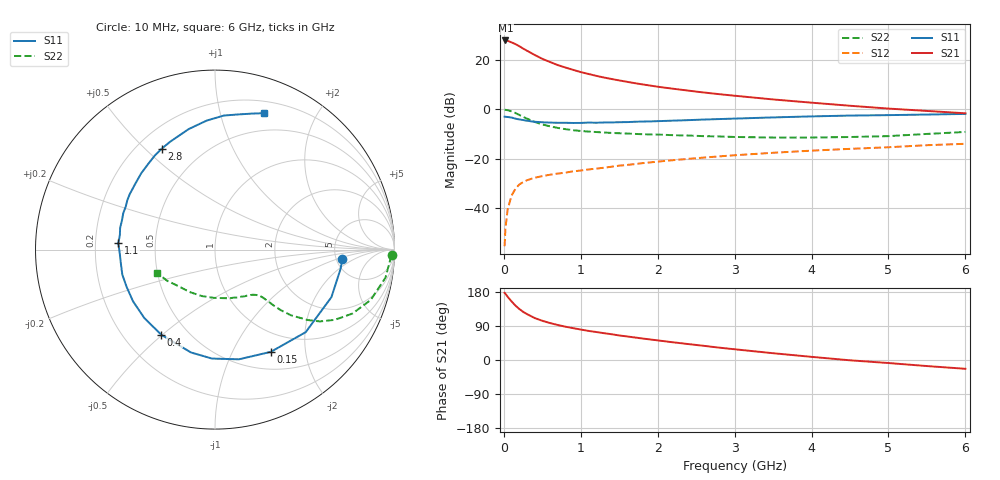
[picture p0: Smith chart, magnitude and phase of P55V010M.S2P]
! SIEMENS Small Signal Semiconductors
! BFP183
! Si NPN RF Bipolar Junction Transistor in SOT143
! VCE = 5 V  IC = 10 mA
! Common Emitter S-Parameters:  March  1996
# GHz  S  MA  R  50
!  f  S11  S21  S12  S22
! GHz  MAG  ANG  MAG  ANG  MAG  ANG  MAG  ANG
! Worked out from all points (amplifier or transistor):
!   36 points, 10 MHz to 6 GHz, reference 50 ohm
!   highest |S21| = 27.9 dB at 20 MHz (marker M1)
!   |S21| within 3 dB of that: start of sweep to 235.8 MHz
!   unconditionally stable (mu >= 1): 1.19 GHz to 5.628 GHz
!   at 250 MHz: K = 0.31, MSG = 27.0 dB, |S12| = -29.5 dB
!   at 1.4 GHz: K = 1.06, MAG = 16.2 dB, |S12| = -23.2 dB
!   at 6 GHz: K = 0.95, MSG = 6.2 dB, |S12| = -13.9 dB
!   lowest NFmin = 1.30 dB at 450 MHz
!   S11 on the Smith chart (normalised r, x): 10 MHz: 5.69, -1.20; 150 MHz: 0.72, -1.42; 400 MHz: 0.36, -0.50; 1.1 GHz: 0.30, +0.03; 2.8 GHz: 0.30, +0.56; 6 GHz: 0.31, +1.38
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0.01  0.7122 -4.2  24.79 177.2  0.0017 88.8  0.9845 -1.9
0.02  0.7074 -8.9  24.82 174.9  0.0038 86.0  0.9766 -3.7
0.05  0.7007 -22.2  24.45 166.7  0.0095 83.0  0.9629 -9.3
0.1  0.6834 -42.3  22.7 154.8  0.0179 70.4  0.9121 -17.9
0.15  0.649 -61.4  21 143.7  0.0246 62.6  0.8441 -25.0
0.2  0.6256 -77.7  19.03 134.8  0.0301 57.5  0.7734 -30.4
0.25  0.6074 -91.6  17.03 127.2  0.0336 52.6  0.7083 -34.4
0.3  0.5884 -103.2  15.43 121.2  0.0367 49.1  0.649 -37.2
0.4  0.5609 -122.3  12.65 110.8  0.0412 44.5  0.5585 -40.9
0.5  0.5481 -136.0  10.54 103.5  0.0445 42.6  0.4959 -42.7
0.6  0.54 -147.8  9.105 97.5  0.0475 41.4  0.453 -43.6
0.7  0.5344 -157.2  7.888 92.4  0.0501 41.5  0.4208 -44.1
0.9  0.53 -171.7  6.311 84.1  0.0557 41.6  0.379 -45.0
1.1  0.5399 176.3  5.208 76.8  0.0607 42.4  0.3549 -46.2
1.5  0.5498 158.5  3.853 64.8  0.0725 43.1  0.3282 -50.0
1.8  0.5667 147.0  3.206 56.8  0.0814 43.3  0.3138 -54.3
2.2  0.5912 134.1  2.615 46.7  0.0936 42.1  0.3001 -61.0
2.8  0.6361 117.7  2.03 32.6  0.1117 39.0  0.2829 -73.6
3.5  0.687 102.4  1.588 17.9  0.1322 34.8  0.269 -91.4
4.5  0.7486 86.2  1.183 -0.8  0.1586 27.6  0.2755 -121.1
5.5  0.7853 74.8  0.929 -16.0  0.1882 20.9  0.3181 -146.9
6  0.8084 70.1  0.833 -23.2  0.201 16.6  0.3493 -158.5
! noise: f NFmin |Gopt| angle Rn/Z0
0.45  1.3  0.15  45  0.18
0.9  1.4  0.2  125  0.19
1.8  2.1  0.34  -170  0.14
